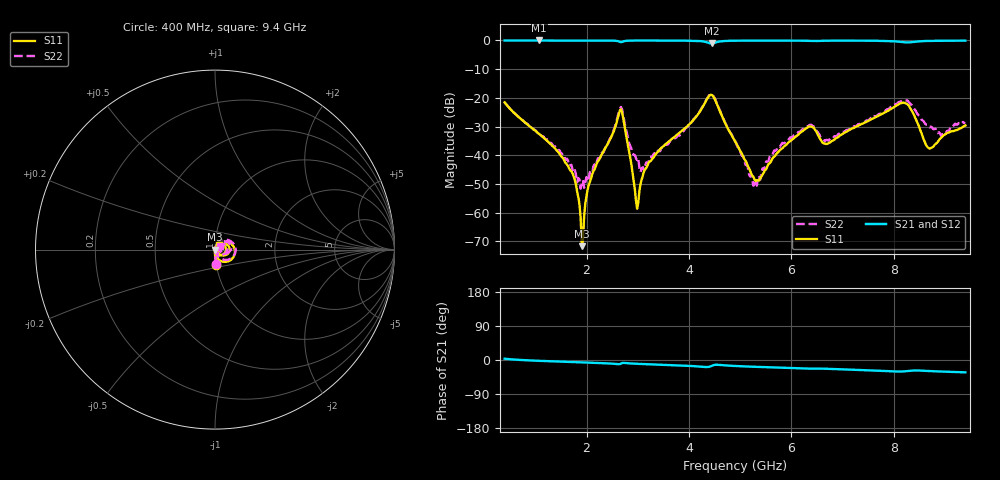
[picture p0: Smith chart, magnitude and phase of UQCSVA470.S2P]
!  Part Number  UQCSVA470  Mounting Orientation: Horizontal
!  Description: Ultra Low ESR Microwave capacitors
!  Application: Coupling, Bypass, Tuning, DC Block
!  Filters, Matching
# GHZ S DB R 50
! Freq  |S11|  S11 Ph  |S21|  S21 Ph  |S12|  S12 Ph  |S22|  S22 Ph
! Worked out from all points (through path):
!   401 points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, 400 MHz to 9.4 GHz, reference 50 ohm
!   highest |S21| = -0.02 dB at 1.075 GHz (marker M1); lowest = -1.1 dB at 4.45 GHz (marker M2)
!   group delay of S21, straight-line fit = 10.2 ps
!   lowest |S11| = -71.7 dB at 1.908 GHz (marker M3), VSWR 1.00, Z = 50 - j0.0181 ohm
!   |S11| at or under -10 dB: start of sweep to end of sweep
!   |S22| runs from -51.7 to -18.7 dB; largest |S21 - S12| = 0.0031
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0.4  -21.59 -85.8  -0.05 3.4  -0.04 3.4  -21.61 -85.0
1.075  -32.60 -91.3  -0.02 -2.2  -0.01 -2.2  -32.29 -86.0
1.728  -46.35 -94.7  -0.02 -5.5  -0.01 -5.5  -45.21 -72.3
1.818  -52.78 -103.0  -0.03 -5.9  -0.01 -5.9  -49.46 -49.3
1.908  -71.69 -135.9  -0.03 -6.3  -0.01 -6.3  -49.62 -7.6
2.088  -48.11 83.2  -0.03 -7.2  -0.02 -7.2  -46.21 32.4
2.65  -24.45 19.1  -0.50 -10.8  -0.49 -10.8  -23.77 21.9
2.718  -27.26 -46.5  -0.37 -7.6  -0.36 -7.7  -26.02 -36.5
2.988  -58.64 -174.2  -0.05 -10.0  -0.04 -10.1  -41.68 -18.6
3.1  -47.10 64.1  -0.05 -10.6  -0.04 -10.7  -44.21 19.1
3.415  -38.42 73.9  -0.04 -12.2  -0.04 -12.3  -38.58 54.4
4.45  -19.05 -21.3  -1.07 -15.1  -1.07 -15.1  -18.85 -10.1
4.9  -35.20 -86.4  -0.10 -15.8  -0.10 -15.9  -34.96 -69.7
5.283  -48.52 -40.0  -0.07 -17.9  -0.07 -18.1  -48.65 -1.9
5.71  -39.52 42.6  -0.07 -19.9  -0.07 -20.0  -38.20 65.5
6.408  -30.11 8.5  -0.23 -22.7  -0.23 -22.9  -29.73 27.3
6.7  -36.06 19.5  -0.10 -23.2  -0.10 -23.3  -34.66 33.6
7.915  -24.25 31.3  -0.22 -29.6  -0.23 -29.7  -23.68 43.9
8.253  -22.09 -12.4  -0.70 -29.3  -0.70 -29.4  -20.87 4.0
8.703  -37.73 -2.5  -0.16 -29.2  -0.17 -29.3  -30.33 -12.6
8.973  -33.08 38.7  -0.13 -30.6  -0.14 -30.7  -32.58 12.7
9.4  -29.65 49.1  -0.09 -32.6  -0.10 -32.7  -28.84 32.0
